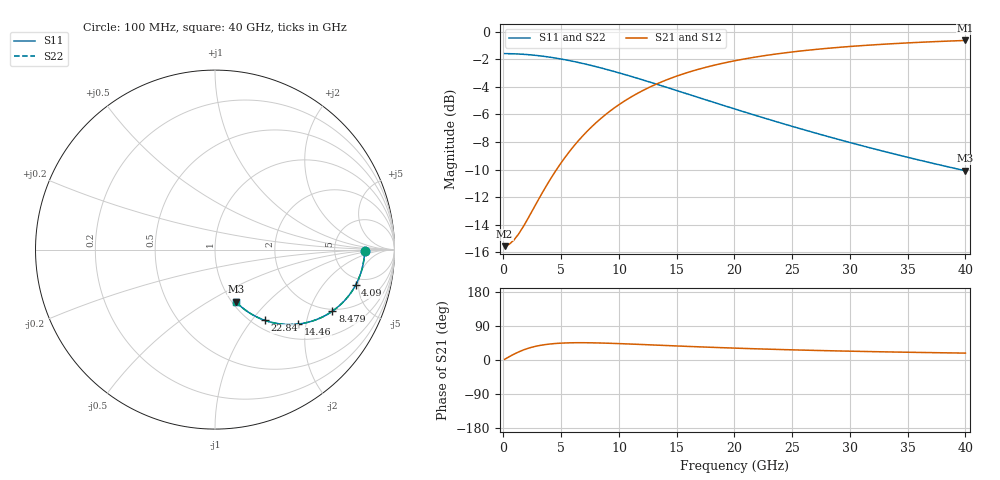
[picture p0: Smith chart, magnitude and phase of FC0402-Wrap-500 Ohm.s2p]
!Vishay Thin-Film
!FC Family
!Case Size 0402
!Assembly Style Full Wrap SMT
!10/21/2015
!thinfilm@vishay.com
# GHz S MA R 50
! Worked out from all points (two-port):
!   101 points, 100 MHz to 40 GHz, reference 50 ohm
!   highest |S21| = -0.63 dB at 40 GHz (marker M1); lowest = -15.6 dB at 100 MHz (marker M2)
!   |S21| within 3 dB of the highest: 13.71 GHz to end of sweep
!   lowest |S11| = -10.1 dB at 40 GHz (marker M3), VSWR 1.91, Z = 52.1 - j33.6 ohm
!   |S11| at or under -10 dB: 39.55 GHz to end of sweep
!   |S22| runs from -10.1 to -1.6 dB; largest |S21 - S12| = 0
!   S11 on the Smith chart (normalised r, x): 100 MHz: 11, -0; 4.09 GHz: 4.04, -4.60; 8.479 GHz: 1.92, -2.89; 14.46 GHz: 1.33, -1.81; 22.84 GHz: 1.13, -1.17; 40 GHz: 1.04, -0.67
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0.1  0.8333 -0.4  0.1668 1.8  0.1668 1.8  0.8333 -0.4
0.499  0.8329 -1.8  0.1694 8.7  0.1694 8.7  0.8329 -1.8
0.898  0.8321 -3.2  0.1754 15.2  0.1754 15.2  0.8321 -3.2
1.297  0.8307 -4.6  0.1843 21.1  0.1843 21.1  0.8307 -4.6
2.494  0.8237 -8.7  0.2241 34.0  0.2241 34.0  0.8237 -8.7
4.09  0.8081 -14.2  0.2931 42.4  0.2931 42.4  0.8081 -14.2
5.287  0.7924 -18.1  0.3482 44.9  0.3482 44.9  0.7924 -18.1
6.085  0.7804 -20.6  0.3845 45.5  0.3845 45.5  0.7804 -20.6
6.883  0.7673 -23.0  0.4198 45.6  0.4198 45.6  0.7673 -23.0
8.479  0.7388 -27.6  0.4865 44.8  0.4865 44.8  0.7388 -27.6
9.676  0.716 -30.9  0.5322 43.6  0.5322 43.6  0.716 -30.9
10.873  0.6925 -33.9  0.5741 42.2  0.5741 42.2  0.6925 -33.9
12.07  0.6689 -36.7  0.6122 40.8  0.6122 40.8  0.6689 -36.7
13.666  0.6377 -40.2  0.6574 38.7  0.6574 38.7  0.6377 -40.2
14.464  0.6224 -41.8  0.6777 37.7  0.6777 37.7  0.6224 -41.8
17.257  0.5711 -46.9  0.7383 34.4  0.7383 34.4  0.5711 -46.9
20.05  0.5245 -51.1  0.7854 31.3  0.7854 31.3  0.5245 -51.1
22.843  0.4828 -54.8  0.8221 28.7  0.8221 28.7  0.4828 -54.8
26.833  0.4314 -59.0  0.8614 25.4  0.8614 25.4  0.4314 -59.0
30.025  0.3963 -61.8  0.8847 23.3  0.8847 23.3  0.3963 -61.8
33.616  0.3623 -64.5  0.9049 21.2  0.9049 21.2  0.3623 -64.5
40  0.3132 -68.2  0.9303 18.2  0.9303 18.2  0.3132 -68.2
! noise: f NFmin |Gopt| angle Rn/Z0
0.1  -4.339e-15  1  0  9.986
4.489  2.893e-15  1  1.542e-15  2.658
8.878  9.643e-16  1  -3.731e-15  0.8451
13.27  -4.822e-16  1  4.812e-15  0.3951
17.66  0  1  1.268e-14  0.2255
22.05  0  1  8.327e-15  0.1446
26.43  0  1  2.43e-14  0.1
30.82  0  1  -1.207e-06  0.07289
35.21  5.051e-09  1  -4.327e-15  0.05519
40  0  1  -1.636e-14  0.04212
